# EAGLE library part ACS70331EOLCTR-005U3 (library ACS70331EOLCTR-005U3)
High Sensitivity, Gmr-Based Current Sensor IC Source: Datasheet
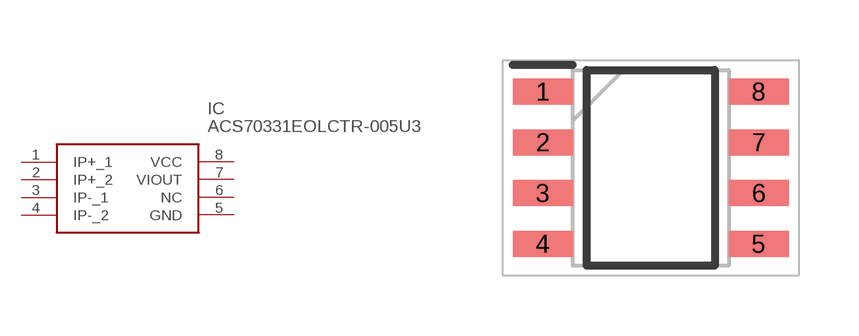
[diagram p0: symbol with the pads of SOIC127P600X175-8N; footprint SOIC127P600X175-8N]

Designator prefix IC

## ACS70331EOLCTR-005U3 (Description: High Sensitivity, Gmr-Based Current Sensor IC; Height: 1.75mm; Manufacturer_Name: Allegro Microsystems; Manufacturer_Part_Number: ACS70331EOLCTR-005U3; Mouser_Part_Number: 250-70331EOLCTR005U3; Mouser_Price-Stock: https://www.mouser.co.uk/ProductDetail/Allegro-MicroSystems/ACS70331EOLCTR-005U3?qs=pUKx8fyJudDz9FJ7uQ14Rw%3D%3D)  [SOIC127P600X175-8N]
1  IP+_1
2  IP+_2
3  IP-_1
4  IP-_2
5  GND
6  NC  nc
7  VIOUT
8  VCC

## Footprint SOIC127P600X175-8N (pad centres in mm)
Package OL, 8-Lead SOIC
smd 1.5 x 0.65: 1 -2.7,1.905; 2 -2.7,0.635; 3 -2.7,-0.635; 4 -2.7,-1.905; 5 2.7,-1.905; 6 2.7,-0.635; 7 2.7,0.635; 8 2.7,1.905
